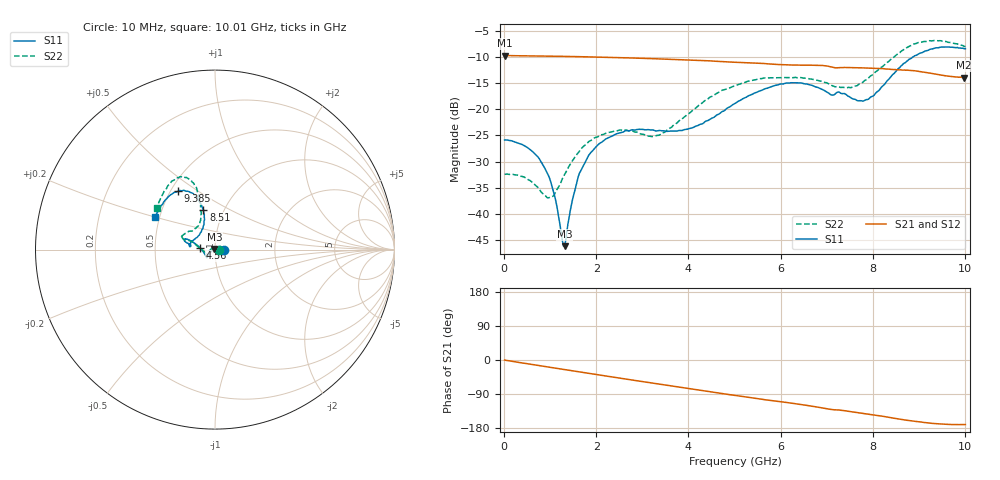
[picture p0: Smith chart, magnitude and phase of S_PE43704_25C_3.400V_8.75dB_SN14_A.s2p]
! Device ID: PE43704
! Dir: z:\PE43704\PE43704_Char_1_20130516\PE43704\AMB\3p400V\8p75dB
! Serial: 14
! Insertion: A
! Impedance: 50 ohm
! Temp: Amb
! VDD: 3.400V
! Attenuation Step: 8.75dB
! IDD: 1.139878e-01mA
#  Hz  S  RI  R  50
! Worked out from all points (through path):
!   401 points, 10 MHz to 10.01 GHz, reference 50 ohm
!   highest |S21| = -9.76 dB at 10 MHz (marker M1); lowest = -14.0 dB at 9.985 GHz (marker M2)
!   group delay of S21, straight-line fit = 49.1 ps
!   lowest |S11| = -46.1 dB at 1.31 GHz (marker M3), VSWR 1.01, Z = 49.7 + j0.367 ohm
!   |S11| at or under -10 dB: start of sweep to 8.877 GHz
!   |S22| runs from -36.9 to -6.9 dB; largest |S21 - S12| = 0.0024
!   S11 on the Smith chart (normalised r, x): 10 MHz: 1.11, +0.00; 4.56 GHz: 0.85, +0.02; 8.51 GHz: 0.80, +0.38; 9.385 GHz: 0.54, +0.42; 10.01 GHz: 0.47, +0.20
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1e7  0.0508 0.000211  0.3253 -0.00124  0.3252 -0.00113  0.0239 0.000258
4.35e8  0.0431 0.013  0.319 -0.0477  0.3194 -0.0478  0.0178 0.0139
8.1e8  0.0261 0.0167  0.3095 -0.0869  0.3095 -0.0869  0.00323 0.0158
1.035e9  0.0132 0.0131  0.3016 -0.1095  0.3015 -0.1093  -0.00896 0.0116
1.26e9  -0.000118 0.00571  0.2912 -0.1316  0.2913 -0.1314  -0.0212 0.00394
1.31e9  -0.00327 0.00369  0.2886 -0.1361  0.2887 -0.1361  -0.0237 0.00146
1.51e9  -0.0143 -0.00512  0.2779 -0.1542  0.278 -0.1542  -0.0326 -0.0079
1.685e9  -0.0233 -0.0137  0.2676 -0.1696  0.2677 -0.1694  -0.0393 -0.0167
2.26e9  -0.0396 -0.0358  0.2278 -0.2139  0.2279 -0.2136  -0.0482 -0.0357
3.36e9  -0.0489 -0.0391  0.1343 -0.2707  0.1347 -0.2705  -0.0539 -0.0169
4.01e9  -0.0635 -0.0149  0.0735 -0.2855  0.0738 -0.2856  -0.0901 0.0122
4.56e9  -0.0835 0.00978  0.0216 -0.2866  0.0223 -0.2867  -0.1287 0.0447
5.01e9  -0.1089 0.0317  -0.0166 -0.2801  -0.0164 -0.2801  -0.1598 0.0513
5.96e9  -0.1612 0.0596  -0.0892 -0.2515  -0.0881 -0.2518  -0.1876 0.0684
6.685e9  -0.1635 0.0418  -0.1396 -0.2228  -0.1394 -0.2226  -0.1737 0.0846
7.36e9  -0.1355 0.0393  -0.1715 -0.1817  -0.1712 -0.1818  -0.112 0.1168
7.76e9  -0.0912 0.0782  -0.1913 -0.158  -0.1907 -0.1585  -0.0819 0.1583
8.36e9  -0.0599 0.1866  -0.2117 -0.1149  -0.2108 -0.1161  -0.0843 0.2774
8.51e9  -0.0642 0.2224  -0.2151 -0.1015  -0.2139 -0.1033  -0.0929 0.3152
9.385e9  -0.2068 0.3256  -0.2107 -0.0443  -0.2109 -0.0439  -0.2242 0.3907
9.985e9  -0.3273 0.189  -0.1978 -0.0333  -0.1992 -0.0333  -0.3191 0.2375
1.001e10  -0.3328 0.1789  -0.1989 -0.0336  -0.2005 -0.0341  -0.3224 0.2296
